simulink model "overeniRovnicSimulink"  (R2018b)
settings: Solver=ode4  StartTime=0.0  StopTime=5  FixedStep=1e-3  RelTol=1e-3
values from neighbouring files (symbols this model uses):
  b_0 = 0    [mainSkript_overeniRovnic.m]    (also in mainSkript_rovniceSystemu.m = (params.bp_0 + params.bn_0) / 2; mainSkript_simulaceLQG.m = (bn_0 + bp_0) / 2; mainSkript_LQGexperiment.m = (bn_0 + bp_0) / 2; mainSkript_LQGexperiment_integral.m = (bn_0 + bp_0) / 2)
  b_1 = params.b_1    [mainSkript_overeniRovnic.m]    (also in mainSkript_rovniceSystemu.m; mainSkript_kyvadlaNajednouOdhad.m; mainSkript_simulaceLQG.m; mainSkript_LQGexperiment.m)
  b_2 = params.b_2    [mainSkript_overeniRovnic.m]    (also in mainSkript_rovniceSystemu.m; mainSkript_kyvadlaNajednouOdhad.m; mainSkript_simulaceLQG.m; mainSkript_LQGexperiment.m)
  dtheta0_0 = 0    [mainSkript_overeniRovnic.m]
  dtheta0_1 = 0    [mainSkript_overeniRovnic.m]    (also in mainSkript_kyvadlaNajednouOdhad.m = filt * dth1(n_start-gl : n_start+gl))
  dtheta0_2 = 0    [mainSkript_overeniRovnic.m]    (also in mainSkript_kyvadlaNajednouOdhad.m = filt * dth2(n_start-gl : n_start+gl))
  g = 9.81    [mainSkript_overeniRovnic.m]    (also in mainSkript_rovniceSystemu.m; mainSkript_estimaceVozik.m; mainSkript_odhadKyvadlaZvlast.m; mainSkript_kyvadlaNajednouOdhad.m)
  I_1 = params.I_1    [mainSkript_overeniRovnic.m]    (also in mainSkript_rovniceSystemu.m; mainSkript_kyvadlaNajednouOdhad.m; mainSkript_simulaceLQG.m; mainSkript_LQGexperiment.m)
  I_2 = params.I_2    [mainSkript_overeniRovnic.m]    (also in mainSkript_rovniceSystemu.m; mainSkript_kyvadlaNajednouOdhad.m; mainSkript_simulaceLQG.m; mainSkript_LQGexperiment.m)
  L_1 = params.L_1    [mainSkript_overeniRovnic.m]    (also in mainSkript_rovniceSystemu.m; odhadovane_parametry.m = 0.228; mainSkript_kyvadlaNajednouOdhad.m; mainSkript_simulaceLQG.m)
  l_1 = params.l_1    [mainSkript_overeniRovnic.m]    (also in mainSkript_rovniceSystemu.m; odhadovane_parametry.m = 0.134; mainSkript_kyvadlaNajednouOdhad.m; mainSkript_simulaceLQG.m)
  l_2 = params.l_2    [mainSkript_overeniRovnic.m]    (also in mainSkript_rovniceSystemu.m; odhadovane_parametry.m = 0.112; mainSkript_kyvadlaNajednouOdhad.m; mainSkript_simulaceLQG.m)
  m = params.m_0    [mainSkript_estimaceVozik.m]    (also in mainSkript_odhadKyvadlaZvlast.m = params.m_2; mainSkript_modifikaceVozik.m = 1.437)
  m_0 = params.m_0    [mainSkript_overeniRovnic.m]    (also in mainSkript_rovniceSystemu.m; mainSkript_simulaceLQG.m; mainSkript_LQGexperiment.m; mainSkript_LQGexperiment_integral.m)
  m_1 = params.m_1    [mainSkript_overeniRovnic.m]    (also in mainSkript_rovniceSystemu.m; mainSkript_kyvadlaNajednouOdhad.m; mainSkript_simulaceLQG.m; mainSkript_LQGexperiment.m)
  m_2 = params.m_2    [mainSkript_overeniRovnic.m]    (also in mainSkript_rovniceSystemu.m; mainSkript_kyvadlaNajednouOdhad.m; mainSkript_simulaceLQG.m; mainSkript_LQGexperiment.m)
  N = N * Cref'    [mainSkript_simulaceLQG.m]    (also in mainSkript_tvorbaTrajektorii.m = 100; mainSkript_pocitaniTVLQR_simplified.m = floor( length(time) / krok ))
  theta0_0 = 0    [mainSkript_overeniRovnic.m]
  theta0_1 = 0.1    [mainSkript_overeniRovnic.m]
  theta0_2 = -0.6    [mainSkript_overeniRovnic.m]
undefined symbols (not defined in the file or in its folder): deg, DiscIntNeverNeededParam, kg, rad, s
libraries: mblibv1 x33, simulink x2
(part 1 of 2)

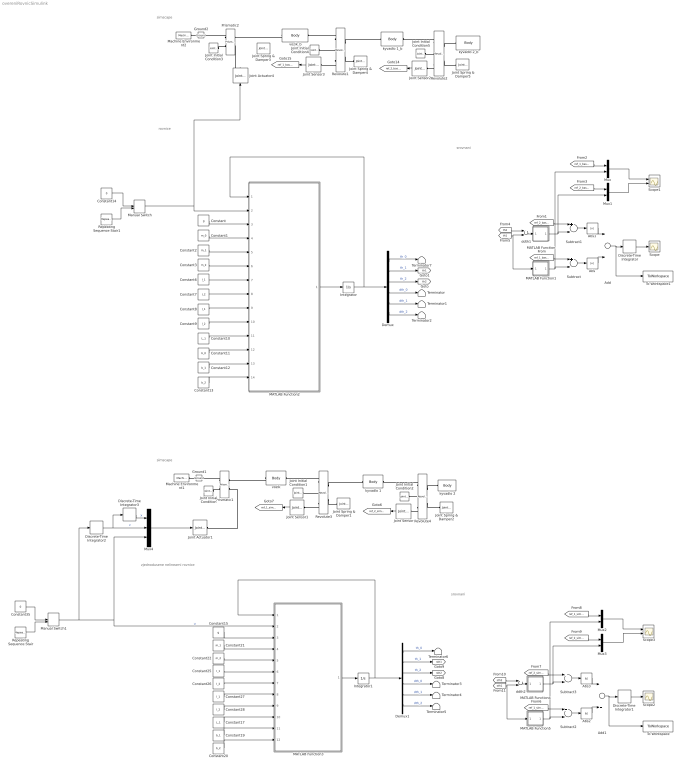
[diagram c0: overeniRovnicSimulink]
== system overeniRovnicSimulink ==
  note: zjednodusene nelinearni rovnice
  note: rovnice
  note: simscape
  note: srovnani
  note: srovnani
  note: simscape
  Abs{,1..3} (4 alike) : Abs
  Add : Sum
  Add1 : Sum
  Constant : Constant  Value=g
  Constant1 : Constant  Value=m_0
  Constant10 : Constant  Value=L_1
  Constant11 : Constant  Value=b_0
  Constant12 : Constant  Value=b_1
  Constant13 : Constant  Value=b_2
  Constant14 : Constant  Value=0
  Constant15 : Constant  Value=g
  Constant17 : Constant  Value=L_1
  Constant19 : Constant  Value=b_1
  Constant2 : Constant  Value=m_1
  Constant20 : Constant  Value=b_2
  Constant21 : Constant  Value=m_1
  Constant22 : Constant  Value=m_2
  Constant25 : Constant  Value=I_1
  Constant26 : Constant  Value=I_2
  Constant27 : Constant  Value=l_1
  Constant28 : Constant  Value=l_2
  Constant3 : Constant  Value=m_2
  Constant35 : Constant  Value=0
  Constant6 : Constant  Value=I_1
  Constant7 : Constant  Value=I_2
  Constant8 : Constant  Value=l_1
  Constant9 : Constant  Value=l_2
  Demux : Demux  Outputs=6
  Demux1 : Demux  Outputs=6
  Discrete-Time Integrator{,1..3} (4 alike) : DiscreteIntegrator  SampleTime=1e-3  ICPrevOutput=DiscIntNeverNeededParam  ICPrevScaledInput=DiscIntNeverNeededParam
  Ground1 : mblibv1/Bodies/Ground  UpdateFromCAD=off  LeftPortType=env  RightPortType=workingframe  PhysicalDomain=Mechanical  DialogClass=GroundBlock  CoordPosition=[0 0 0]  CoordPositionUnits=m  StateVectorMgrId=-1  MachineId=[0 0]  ShowEnvPort=on  ParameterChecksum=[1731498079, 3636340835, 3655824204, 100592062]  TopologyChecksum=[3274135082, 1712955816, 1157478112, 3607701974]
  Ground2 : mblibv1/Bodies/Ground  UpdateFromCAD=off  LeftPortType=env  RightPortType=workingframe  PhysicalDomain=Mechanical  DialogClass=GroundBlock  CoordPosition=[0 0 0]  CoordPositionUnits=m  StateVectorMgrId=-1  MachineId=[0 0]  ShowEnvPort=on  ParameterChecksum=[3763866834, 2337324317, 1522709240, 4291601322]  TopologyChecksum=[3204540527, 4191976194, 257722546, 2930277444]
  Integrator : Integrator  InitialCondition=[theta0_0, theta0_1, theta0_2, dtheta0_0, dtheta0_1, dtheta0_2]
  Integrator1 : Integrator  InitialCondition=[theta0_0, theta0_1, theta0_2, dtheta0_0, dtheta0_1, dtheta0_2]
  Joint Actuator1 : mblibv1/Sensors &  Actuators/Joint Actuator  UpdateFromCAD=off  PhysicalDomain=Mechanical  PortType=blob  ActuationStyle=Motion  AngleUnits=rad  ArcVelocityUnits=rad/s  ArcAccelerationUnits=rad/s^2  CoordPositionUnits=m  VelocityUnits=m/s  AccelerationUnits=m/s^2  ForceUnits=N  TorqueUnits=N*m  ActiveIO=on  Width=3  DialogClass=MechanicalActuatorBlock  Primitive=P1  ReferenceFrame=Absolute (World)
  Joint Actuator4 : mblibv1/Sensors &  Actuators/Joint Actuator  UpdateFromCAD=off  PhysicalDomain=Mechanical  PortType=blob  ActuationStyle=Force  AngleUnits=rad  ArcVelocityUnits=rad/s  ArcAccelerationUnits=rad/s^2  CoordPositionUnits=m  VelocityUnits=m/s  AccelerationUnits=m/s^2  ForceUnits=N  TorqueUnits=N*m  ActiveIO=on  Width=1  DialogClass=MechanicalActuatorBlock  Primitive=P1  ReferenceFrame=Absolute (World)
  Joint Initial Condition : mblibv1/Sensors &  Actuators/Joint Initial Condition  UpdateFromCAD=off  LeftPortType=blob  RightPortType=blob  PhysicalDomain=mechanical  DialogClass=InitialConditionBlock  InitialConditions=P1$true$theta0_0$m$deg$dtheta0_0$m/s$deg/s#P2$false$0$m$deg$0$m/s$deg/s#P3$false$0$m$deg$0$m/s$deg/s#R1$false$0$m$deg$0$m/s$deg/s#R2$false$0$m$deg$0$m/s$deg/s#R3$false$0$m$deg$0$m/s$deg/s#S$false$0$m$deg$0$m/s$deg/s  P1PIC=theta0_0  P1VIC=dtheta0_0  P2PIC=0  P2VIC=0  P3PIC=0  P3VIC=0  R1PIC=0  R1VIC=0  R2PIC=0  R2VIC=0  R3PIC=0  R3VIC=0  SPIC=0  SVIC=0
  Joint Initial Condition1 : mblibv1/Sensors &  Actuators/Joint Initial Condition  UpdateFromCAD=off  LeftPortType=blob  RightPortType=blob  PhysicalDomain=mechanical  DialogClass=InitialConditionBlock  InitialConditions=P1$false$th0i$m$deg$dth0i$m/s$deg/s#P2$false$0$m$deg$0$m/s$deg/s#P3$false$0$m$deg$0$m/s$deg/s#R1$true$theta0_1$m$rad$dtheta0_1$m/s$rad/s#R2$false$0$m$deg$0$m/s$deg/s#R3$false$0$m$deg$0$m/s$deg/s#S$false$0$m$deg$0$m/s$deg/s  P1PIC=0  P1VIC=0  P2PIC=0  P2VIC=0  P3PIC=0  P3VIC=0  R1PIC=theta0_1  R1VIC=dtheta0_1  R2PIC=0  R2VIC=0  R3PIC=0  R3VIC=0  SPIC=0  SVIC=0
  Joint Initial Condition2 : mblibv1/Sensors &  Actuators/Joint Initial Condition  UpdateFromCAD=off  LeftPortType=blob  RightPortType=blob  PhysicalDomain=mechanical  DialogClass=InitialConditionBlock  InitialConditions=P1$false$th0i$m$deg$dth0i$m/s$deg/s#P2$false$0$m$deg$0$m/s$deg/s#P3$false$0$m$deg$0$m/s$deg/s#R1$true$theta0_2 - theta0_1$m$rad$dtheta0_2 - dtheta0_1$m/s$rad/s#R2$false$0$m$deg$0$m/s$deg/s#R3$false$0$m$deg$0$m/s$deg/s#S$false$0$m$deg$0$m/s$deg/s  P1PIC=0  P1VIC=0  P2PIC=0  P2VIC=0  P3PIC=0  P3VIC=0  R1PIC=theta0_2 - theta0_1  R1VIC=dtheta0_2 - dtheta0_1  R2PIC=0  R2VIC=0  R3PIC=0  R3VIC=0  SPIC=0  SVIC=0
  Joint Initial Condition3 : mblibv1/Sensors &  Actuators/Joint Initial Condition  UpdateFromCAD=off  LeftPortType=blob  RightPortType=blob  PhysicalDomain=mechanical  DialogClass=InitialConditionBlock  InitialConditions=P1$true$theta0_0$m$deg$dtheta0_0$m/s$deg/s#P2$false$0$m$deg$0$m/s$deg/s#P3$false$0$m$deg$0$m/s$deg/s#R1$false$0$m$deg$0$m/s$deg/s#R2$false$0$m$deg$0$m/s$deg/s#R3$false$0$m$deg$0$m/s$deg/s#S$false$0$m$deg$0$m/s$deg/s  P1PIC=theta0_0  P1VIC=dtheta0_0  P2PIC=0  P2VIC=0  P3PIC=0  P3VIC=0  R1PIC=0  R1VIC=0  R2PIC=0  R2VIC=0  R3PIC=0  R3VIC=0  SPIC=0  SVIC=0
  Joint Initial Condition4 : mblibv1/Sensors &  Actuators/Joint Initial Condition  UpdateFromCAD=off  LeftPortType=blob  RightPortType=blob  PhysicalDomain=mechanical  DialogClass=InitialConditionBlock  InitialConditions=P1$false$th0i$m$deg$dth0i$m/s$deg/s#P2$false$0$m$deg$0$m/s$deg/s#P3$false$0$m$deg$0$m/s$deg/s#R1$true$theta0_1$m$rad$dtheta0_1$m/s$rad/s#R2$false$0$m$deg$0$m/s$deg/s#R3$false$0$m$deg$0$m/s$deg/s#S$false$0$m$deg$0$m/s$deg/s  P1PIC=0  P1VIC=0  P2PIC=0  P2VIC=0  P3PIC=0  P3VIC=0  R1PIC=theta0_1  R1VIC=dtheta0_1  R2PIC=0  R2VIC=0  R3PIC=0  R3VIC=0  SPIC=0  SVIC=0
  Joint Initial Condition5 : mblibv1/Sensors &  Actuators/Joint Initial Condition  UpdateFromCAD=off  LeftPortType=blob  RightPortType=blob  PhysicalDomain=mechanical  DialogClass=InitialConditionBlock  InitialConditions=P1$false$th0i$m$deg$dth0i$m/s$deg/s#P2$false$0$m$deg$0$m/s$deg/s#P3$false$0$m$deg$0$m/s$deg/s#R1$true$theta0_2 - theta0_1$m$rad$dtheta0_2 - dtheta0_1$m/s$rad/s#R2$false$0$m$deg$0$m/s$deg/s#R3$false$0$m$deg$0$m/s$deg/s#S$false$0$m$deg$0$m/s$deg/s  P1PIC=0  P1VIC=0  P2PIC=0  P2VIC=0  P3PIC=0  P3VIC=0  R1PIC=theta0_2 - theta0_1  R1VIC=dtheta0_2 - dtheta0_1  R2PIC=0  R2VIC=0  R3PIC=0  R3VIC=0  SPIC=0  SVIC=0
  Joint Sensor{,1..3} (4 alike) : mblibv1/Sensors &  Actuators/Joint Sensor  UpdateFromCAD=off  PhysicalDomain=Mechanical  PortType=blob  Muxed=on  Pose=off  Angle=on  AngleUnits=rad  ArcVelocity=off  ArcVelocityUnits=deg/s  ArcAcceleration=off  ArcAccelerationUnits=deg/s^2  CoordPosition=on  CoordPositionUnits=m  Velocity=off  VelocityUnits=m/s  Acceleration=off  AccelerationUnits=m/s^2  Quaternion=on  QuaternionDT=off  QuaternionDDT=off  QuaternionUnits=off  OutputVector=[1]  ActiveIO=on  Width=1  DialogClass=MechanicalSensorBlock  Primitive=R1  Force=off  ForceUnits=N  Torque=off  TorqueUnits=N*m  ReferenceFrame=Absolute (World)  ReactionSensedSide=Base  ReactionReferenceFrame=Absolute (World)  ReactionForce=off  ReactionForceUnits=N  ReactionMoment=off  ReactionMomentUnits=N*m
  Joint Spring & Damper1 : mblibv1/Force  Elements/Joint Spring & Damper  UpdateFromCAD=off  DialogClass=JointSpringDamper  JFEParameters=P1$false$0$b0$0$m$m/s$N$deg$deg/s$N*m#P2$false$0$0$0$m$m/s$N$deg$deg/s$N*m#P3$false$0$0$0$m$m/s$N$deg$deg/s$N*m#R1$true$0$b_1$0$m$m/s$N$rad$rad/s$N*m#R2$false$0$0$0$m$m/s$N$deg$deg/s$N*m#R3$false$0$0$0$m$m/s$N$deg$deg/s$N*m#S$false$0$0$0$m$m/s$N$deg$deg/s$N*m
  Joint Spring & Damper2 : mblibv1/Force  Elements/Joint Spring & Damper  UpdateFromCAD=off  DialogClass=JointSpringDamper  JFEParameters=P1$false$0$b0$0$m$m/s$N$deg$deg/s$N*m#P2$false$0$0$0$m$m/s$N$deg$deg/s$N*m#P3$false$0$0$0$m$m/s$N$deg$deg/s$N*m#R1$true$0$b_2$0$m$m/s$N$rad$rad/s$N*m#R2$false$0$0$0$m$m/s$N$deg$deg/s$N*m#R3$false$0$0$0$m$m/s$N$deg$deg/s$N*m#S$false$0$0$0$m$m/s$N$deg$deg/s$N*m
  Joint Spring & Damper3 : mblibv1/Force  Elements/Joint Spring & Damper  UpdateFromCAD=off  DialogClass=JointSpringDamper  JFEParameters=P1$true$0$b_0$0$m$m/s$N$deg$deg/s$N*m#P2$false$0$0$0$m$m/s$N$deg$deg/s$N*m#P3$false$0$0$0$m$m/s$N$deg$deg/s$N*m#R1$false$0$0$0$m$m/s$N$deg$deg/s$N*m#R2$false$0$0$0$m$m/s$N$deg$deg/s$N*m#R3$false$0$0$0$m$m/s$N$deg$deg/s$N*m#S$false$0$0$0$m$m/s$N$deg$deg/s$N*m
  Joint Spring & Damper4 : mblibv1/Force  Elements/Joint Spring & Damper  UpdateFromCAD=off  DialogClass=JointSpringDamper  JFEParameters=P1$false$0$b0$0$m$m/s$N$deg$deg/s$N*m#P2$false$0$0$0$m$m/s$N$deg$deg/s$N*m#P3$false$0$0$0$m$m/s$N$deg$deg/s$N*m#R1$true$0$b_1$0$m$m/s$N$rad$rad/s$N*m#R2$false$0$0$0$m$m/s$N$deg$deg/s$N*m#R3$false$0$0$0$m$m/s$N$deg$deg/s$N*m#S$false$0$0$0$m$m/s$N$deg$deg/s$N*m
  Joint Spring & Damper5 : mblibv1/Force  Elements/Joint Spring & Damper  UpdateFromCAD=off  DialogClass=JointSpringDamper  JFEParameters=P1$false$0$b0$0$m$m/s$N$deg$deg/s$N*m#P2$false$0$0$0$m$m/s$N$deg$deg/s$N*m#P3$false$0$0$0$m$m/s$N$deg$deg/s$N*m#R1$true$0$b_2$0$m$m/s$N$rad$rad/s$N*m#R2$false$0$0$0$m$m/s$N$deg$deg/s$N*m#R3$false$0$0$0$m$m/s$N$deg$deg/s$N*m#S$false$0$0$0$m$m/s$N$deg$deg/s$N*m
  MATLAB Function : MATLAB Function  TreatAsAtomicUnit=on
  MATLAB Function1 : MATLAB Function  TreatAsAtomicUnit=on
  MATLAB Function2 : MATLAB Function  TreatAsAtomicUnit=on
  MATLAB Function3 : MATLAB Function  TreatAsAtomicUnit=on
  MATLAB Function4 : MATLAB Function  TreatAsAtomicUnit=on
  MATLAB Function5 : MATLAB Function  TreatAsAtomicUnit=on
  Machine Environment1 : mblibv1/Bodies/Machine Environment  PortType=env  PhysicalDomain=Mechanical  DialogTemplateClass=MECH.MachineEnvironment  SyncWhenCopied=off  Gravity=[0 -g 0]  GravityUnits=m/s^2  GravityAsSignal=off  Dimensionality=Auto-detect  AnalysisType=Forward dynamics  LinearAssemblyTolerance=1e-3  LinearAssemblyToleranceUnits=m  AngularAssemblyTolerance=1e-3  AngularAssemblyToleranceUnits=rad  ConstraintSolverType=Stabilizing  ConstraintRelTolerance=1e-4  ConstraintAbsTolerance=1e-4  UseRobustSingularityHandling=off  RedundancyAnalysisToleranceType=Automatically select tolerance  RedundancyAnalysisTolerance=1e-14  StatePerturbationType=Fixed  PerturbationSize=1e-5  VisualizeMachine=on  BodyVisualizationType=Use model default body geometries  BodyColorSelMode=Use model default  DefaultBodyColor=[1 0 0]
  Machine Environment2 : mblibv1/Bodies/Machine Environment  PortType=env  PhysicalDomain=Mechanical  DialogTemplateClass=MECH.MachineEnvironment  SyncWhenCopied=off  Gravity=[0 -g 0]  GravityUnits=m/s^2  GravityAsSignal=off  Dimensionality=Auto-detect  AnalysisType=Forward dynamics  LinearAssemblyTolerance=1e-3  LinearAssemblyToleranceUnits=m  AngularAssemblyTolerance=1e-3  AngularAssemblyToleranceUnits=rad  ConstraintSolverType=Stabilizing  ConstraintRelTolerance=1e-4  ConstraintAbsTolerance=1e-4  UseRobustSingularityHandling=off  RedundancyAnalysisToleranceType=Automatically select tolerance  RedundancyAnalysisTolerance=1e-14  StatePerturbationType=Fixed  PerturbationSize=1e-5  VisualizeMachine=on  BodyVisualizationType=Use model default body geometries  BodyColorSelMode=Use model default  DefaultBodyColor=[1 0 0]
  Manual Switch : ManualSwitch  CurrentSetting=0
  Manual Switch1 : ManualSwitch  CurrentSetting=0
  Mux{,1..3} (4 alike) : Mux  Inputs=2
  Mux4 : Mux  Inputs=3
  Prismatic1 : mblibv1/Joints/Prismatic  LConnTagsString=__newl0|SA1  RConnTagsString=__newr0|SA1  UpdateFromCAD=off  NumSAPorts=2  CutJoint=off  MarkAsCut=off  Primitives=prismatic  PrimitiveProps=P1$World$[-1 0 0]$prismatic  DialogClass=JointBlock  P1Axis=[-1 0 0]
  Prismatic2 : mblibv1/Joints/Prismatic  LConnTagsString=__newl0|SA1  RConnTagsString=__newr0|SA1  UpdateFromCAD=off  NumSAPorts=2  CutJoint=off  MarkAsCut=off  Primitives=prismatic  PrimitiveProps=P1$World$[-1 0 0]$prismatic  DialogClass=JointBlock  P1Axis=[-1 0 0]
  Repeating Sequence Stair : simulink/Sources/Repeating Sequence Stair  OutValues=[3 -3 2 -2 0].'  tsamp=-1  OutMin=[]  OutMax=[]  OutDataTypeStr=double  OutputDataTypeScalingMode=double  OutDataType=fixdt(0,8)  ConRadixGroup=Best Precision: Vector-wise  OutScaling=2^-12
  Repeating Sequence Stair1 : simulink/Sources/Repeating Sequence Stair  OutValues=[3 -3 2 -2 0].'  tsamp=-1  OutMin=[]  OutMax=[]  OutDataTypeStr=double  OutputDataTypeScalingMode=double  OutDataType=fixdt(0,8)  ConRadixGroup=Best Precision: Vector-wise  OutScaling=2^-12
  Revolute1 : mblibv1/Joints/Revolute  LConnTagsString=__newl0|SA1|SA2  RConnTagsString=__newr0|SA1  UpdateFromCAD=off  NumSAPorts=3  CutJoint=off  MarkAsCut=off  Primitives=prismatic  PrimitiveProps=R1$World$[0 0 1]$revolute  DialogClass=JointBlock  R1Axis=[0 0 1]
  Revolute2 : mblibv1/Joints/Revolute  LConnTagsString=__newl0|SA1|SA2  RConnTagsString=__newr0|SA1  UpdateFromCAD=off  NumSAPorts=3  CutJoint=off  MarkAsCut=off  Primitives=prismatic  PrimitiveProps=R1$Base$[0 0 1]$revolute  DialogClass=JointBlock  R1Axis=[0 0 1]
  Revolute3 : mblibv1/Joints/Revolute  LConnTagsString=__newl0|SA1|SA2  RConnTagsString=__newr0|SA1  UpdateFromCAD=off  NumSAPorts=3  CutJoint=off  MarkAsCut=off  Primitives=prismatic  PrimitiveProps=R1$World$[0 0 1]$revolute  DialogClass=JointBlock  R1Axis=[0 0 1]
  Revolute4 : mblibv1/Joints/Revolute  LConnTagsString=__newl0|SA1|SA2  RConnTagsString=__newr0|SA1  UpdateFromCAD=off  NumSAPorts=3  CutJoint=off  MarkAsCut=off  Primitives=prismatic  PrimitiveProps=R1$Base$[0 0 1]$revolute  DialogClass=JointBlock  R1Axis=[0 0 1]
  Scope : Scope
  Scope1 : Scope  NumInputPorts=2
  Scope2 : Scope
  Scope3 : Scope  NumInputPorts=2
  Subtract{,1..3} (4 alike) : Sum  Inputs=+-
  Terminator{,1..7} (8 alike) : Terminator
  To Workspace : ToWorkspace  VariableName=odchylka_simplified  SaveFormat=Structure With Time  SampleTime=-1
  To Workspace1 : ToWorkspace  VariableName=odchylka_basic  SaveFormat=Structure With Time  SampleTime=-1
  ddth1 : Sum  Inputs=+-
  ddth2 : Sum  Inputs=+-
  kyvadlo 1 : mblibv1/Bodies/Body  LConnTagsString=CS1  RConnTagsString=CS2  UpdateFromCAD=off  DialogClass=MechanicalBodyBlock  Mass=m_1  MassUnits=kg  InertiaUnits=kg*m^2  Inertia=eye(3)*I_1  Shape=Cylinder  ShapeDims=[1 1]  ShapeUnits=m  ShapeUse=false  Density=1  DensityUnits=kg/m^3  DensityUse=false  GraphicsMode=MACHINE_DEFAULT  BodyColorSelMode=COLORPALETTE  BodyColor=[0 0 0]  AttachedToCS=CG  CG=Left$CG$[0 l_1 0]$CS1$CS1$m$[0 0 0]$Euler X-Y-Z$deg$WORLD$false$none  WorkingFrames=Left$CS1$[0 0 0]$Adjoining$Adjoining$m$[0 0 0]$Euler X-Y-Z$deg$WORLD$true$none#Right$CS2$[0 L_1 0]$CS1$CS1$m$[0 0 0]$Euler X-Y-Z$deg$WORLD$true$none  CGPos=[0 l_1 0]  CGRot=[0 0 0]  CS0Pos=[]  CS0Rot=[]  CS1Pos=[0 0 0]  CS1Rot=[0 0 0]  CS2Pos=[0 L_1 0]  CS2Rot=[0 0 0]  CS3Pos=[]  CS3Rot=[]  CS4Pos=[]  CS4Rot=[]  CS5Pos=[]  CS5Rot=[]  CS6Pos=[]  CS6Rot=[]  CS7Pos=[]  CS7Rot=[]  CS8Pos=[]  CS8Rot=[]  CS9Pos=[]  CS9Rot=[]  CS10Pos=[]  CS10Rot=[]  CS11Pos=[]  CS11Rot=[]  CS12Pos=[]  CS12Rot=[]  CS13Pos=[]  CS13Rot=[]  CS14Pos=[]  CS14Rot=[]  CS15Pos=[]  CS15Rot=[]  CS16Pos=[]  CS16Rot=[]  CS17Pos=[]  CS17Rot=[]  CS18Pos=[]  CS18Rot=[]  CS19Pos=[]  CS19Rot=[]  CS20Pos=[]  CS20Rot=[]
  kyvadlo 1_b : mblibv1/Bodies/Body  LConnTagsString=CS1  RConnTagsString=CS2  UpdateFromCAD=off  DialogClass=MechanicalBodyBlock  Mass=m_1  MassUnits=kg  InertiaUnits=kg*m^2  Inertia=eye(3)*I_1  Shape=Cylinder  ShapeDims=[1 1]  ShapeUnits=m  ShapeUse=false  Density=1  DensityUnits=kg/m^3  DensityUse=false  GraphicsMode=MACHINE_DEFAULT  BodyColorSelMode=COLORPALETTE  BodyColor=[0 0 0]  AttachedToCS=CG  CG=Left$CG$[0 l_1 0]$CS1$CS1$m$[0 0 0]$Euler X-Y-Z$deg$WORLD$false$none  WorkingFrames=Left$CS1$[0 0 0]$Adjoining$Adjoining$m$[0 0 0]$Euler X-Y-Z$deg$WORLD$true$none#Right$CS2$[0 L_1 0]$CS1$CS1$m$[0 0 0]$Euler X-Y-Z$deg$WORLD$true$none  CGPos=[0 l_1 0]  CGRot=[0 0 0]  CS0Pos=[]  CS0Rot=[]  CS1Pos=[0 0 0]  CS1Rot=[0 0 0]  CS2Pos=[0 L_1 0]  CS2Rot=[0 0 0]  CS3Pos=[]  CS3Rot=[]  CS4Pos=[]  CS4Rot=[]  CS5Pos=[]  CS5Rot=[]  CS6Pos=[]  CS6Rot=[]  CS7Pos=[]  CS7Rot=[]  CS8Pos=[]  CS8Rot=[]  CS9Pos=[]  CS9Rot=[]  CS10Pos=[]  CS10Rot=[]  CS11Pos=[]  CS11Rot=[]  CS12Pos=[]  CS12Rot=[]  CS13Pos=[]  CS13Rot=[]  CS14Pos=[]  CS14Rot=[]  CS15Pos=[]  CS15Rot=[]  CS16Pos=[]  CS16Rot=[]  CS17Pos=[]  CS17Rot=[]  CS18Pos=[]  CS18Rot=[]  CS19Pos=[]  CS19Rot=[]  CS20Pos=[]  CS20Rot=[]
  kyvadlo 2 : mblibv1/Bodies/Body  LConnTagsString=CS1  RConnTagsString=CS2  UpdateFromCAD=off  DialogClass=MechanicalBodyBlock  Mass=m_2  MassUnits=kg  InertiaUnits=kg*m^2  Inertia=eye(3)*I_2  Shape=Cylinder  ShapeDims=[1 1]  ShapeUnits=m  ShapeUse=false  Density=1  DensityUnits=kg/m^3  DensityUse=false  GraphicsMode=MACHINE_DEFAULT  BodyColorSelMode=COLORPALETTE  BodyColor=[0 0 0]  AttachedToCS=CG  CG=Left$CG$[0 l_2 0]$CS1$CS1$m$[0 0 0]$Euler X-Y-Z$deg$WORLD$false$none  WorkingFrames=Left$CS1$[0 0 0]$Adjoining$Adjoining$m$[0 0 0]$Euler X-Y-Z$deg$WORLD$true$none#Right$CS2$[0 2*l_2 0]$CS1$CS1$m$[0 0 0]$Euler X-Y-Z$deg$WORLD$true$none  CGPos=[0 l_2 0]  CGRot=[0 0 0]  CS0Pos=[]  CS0Rot=[]  CS1Pos=[0 0 0]  CS1Rot=[0 0 0]  CS2Pos=[0 2*l_2 0]  CS2Rot=[0 0 0]  CS3Pos=[]  CS3Rot=[]  CS4Pos=[]  CS4Rot=[]  CS5Pos=[]  CS5Rot=[]  CS6Pos=[]  CS6Rot=[]  CS7Pos=[]  CS7Rot=[]  CS8Pos=[]  CS8Rot=[]  CS9Pos=[]  CS9Rot=[]  CS10Pos=[]  CS10Rot=[]  CS11Pos=[]  CS11Rot=[]  CS12Pos=[]  CS12Rot=[]  CS13Pos=[]  CS13Rot=[]  CS14Pos=[]  CS14Rot=[]  CS15Pos=[]  CS15Rot=[]  CS16Pos=[]  CS16Rot=[]  CS17Pos=[]  CS17Rot=[]  CS18Pos=[]  CS18Rot=[]  CS19Pos=[]  CS19Rot=[]  CS20Pos=[]  CS20Rot=[]
  kyvadlo 2_b : mblibv1/Bodies/Body  LConnTagsString=CS1  RConnTagsString=CS2  UpdateFromCAD=off  DialogClass=MechanicalBodyBlock  Mass=m_2  MassUnits=kg  InertiaUnits=kg*m^2  Inertia=eye(3)*I_2  Shape=Cylinder  ShapeDims=[1 1]  ShapeUnits=m  ShapeUse=false  Density=1  DensityUnits=kg/m^3  DensityUse=false  GraphicsMode=MACHINE_DEFAULT  BodyColorSelMode=COLORPALETTE  BodyColor=[0 0 0]  AttachedToCS=CG  CG=Left$CG$[0 l_2 0]$CS1$CS1$m$[0 0 0]$Euler X-Y-Z$deg$WORLD$false$none  WorkingFrames=Left$CS1$[0 0 0]$Adjoining$Adjoining$m$[0 0 0]$Euler X-Y-Z$deg$WORLD$true$none#Right$CS2$[0 2*l_2 0]$CS1$CS1$m$[0 0 0]$Euler X-Y-Z$deg$WORLD$true$none  CGPos=[0 l_2 0]  CGRot=[0 0 0]  CS0Pos=[]  CS0Rot=[]  CS1Pos=[0 0 0]  CS1Rot=[0 0 0]  CS2Pos=[0 2*l_2 0]  CS2Rot=[0 0 0]  CS3Pos=[]  CS3Rot=[]  CS4Pos=[]  CS4Rot=[]  CS5Pos=[]  CS5Rot=[]  CS6Pos=[]  CS6Rot=[]  CS7Pos=[]  CS7Rot=[]  CS8Pos=[]  CS8Rot=[]  CS9Pos=[]  CS9Rot=[]  CS10Pos=[]  CS10Rot=[]  CS11Pos=[]  CS11Rot=[]  CS12Pos=[]  CS12Rot=[]  CS13Pos=[]  CS13Rot=[]  CS14Pos=[]  CS14Rot=[]  CS15Pos=[]  CS15Rot=[]  CS16Pos=[]  CS16Rot=[]  CS17Pos=[]  CS17Rot=[]  CS18Pos=[]  CS18Rot=[]  CS19Pos=[]  CS19Rot=[]  CS20Pos=[]  CS20Rot=[]
  vozik_b : mblibv1/Bodies/Body  LConnTagsString=CS1  RConnTagsString=CS2  UpdateFromCAD=off  DialogClass=MechanicalBodyBlock  Mass=m_0  MassUnits=kg  InertiaUnits=kg*m^2  Inertia=zeros(3)  Shape=Cylinder  ShapeDims=[1 1]  ShapeUnits=m  ShapeUse=false  Density=1  DensityUnits=kg/m^3  DensityUse=false  GraphicsMode=MACHINE_DEFAULT  BodyColorSelMode=COLORPALETTE  BodyColor=[0 0 0]  AttachedToCS=CG  CG=Left$CG$[0 0 0]$WORLD$WORLD$m$[0 0 0]$Euler X-Y-Z$deg$WORLD$false$none  WorkingFrames=Left$CS1$[0 0 0]$CG$CG$m$[0 0 0]$Euler X-Y-Z$deg$WORLD$true$none#Right$CS2$[0 0 0]$CG$CG$m$[0 0 0]$Euler X-Y-Z$deg$WORLD$true$none  CGPos=[0 0 0]  CGRot=[0 0 0]  CS0Pos=[]  CS0Rot=[]  CS1Pos=[0 0 0]  CS1Rot=[0 0 0]  CS2Pos=[0 0 0]  CS2Rot=[0 0 0]  CS3Pos=[]  CS3Rot=[]  CS4Pos=[]  CS4Rot=[]  CS5Pos=[]  CS5Rot=[]  CS6Pos=[]  CS6Rot=[]  CS7Pos=[]  CS7Rot=[]  CS8Pos=[]  CS8Rot=[]  CS9Pos=[]  CS9Rot=[]  CS10Pos=[]  CS10Rot=[]  CS11Pos=[]  CS11Rot=[]  CS12Pos=[]  CS12Rot=[]  CS13Pos=[]  CS13Rot=[]  CS14Pos=[]  CS14Rot=[]  CS15Pos=[]  CS15Rot=[]  CS16Pos=[]  CS16Rot=[]  CS17Pos=[]  CS17Rot=[]  CS18Pos=[]  CS18Rot=[]  CS19Pos=[]  CS19Rot=[]  CS20Pos=[]  CS20Rot=[]
  vozík : mblibv1/Bodies/Body  LConnTagsString=CS1  RConnTagsString=CS2  UpdateFromCAD=off  DialogClass=MechanicalBodyBlock  Mass=m_0  MassUnits=kg  InertiaUnits=kg*m^2  Inertia=zeros(3)  Shape=Cylinder  ShapeDims=[1 1]  ShapeUnits=m  ShapeUse=false  Density=1  DensityUnits=kg/m^3  DensityUse=false  GraphicsMode=MACHINE_DEFAULT  BodyColorSelMode=COLORPALETTE  BodyColor=[0 0 0]  AttachedToCS=CG  CG=Left$CG$[0 0 0]$WORLD$WORLD$m$[0 0 0]$Euler X-Y-Z$deg$WORLD$false$none  WorkingFrames=Left$CS1$[0 0 0]$CG$CG$m$[0 0 0]$Euler X-Y-Z$deg$WORLD$true$none#Right$CS2$[0 0 0]$CG$CG$m$[0 0 0]$Euler X-Y-Z$deg$WORLD$true$none  CGPos=[0 0 0]  CGRot=[0 0 0]  CS0Pos=[]  CS0Rot=[]  CS1Pos=[0 0 0]  CS1Rot=[0 0 0]  CS2Pos=[0 0 0]  CS2Rot=[0 0 0]  CS3Pos=[]  CS3Rot=[]  CS4Pos=[]  CS4Rot=[]  CS5Pos=[]  CS5Rot=[]  CS6Pos=[]  CS6Rot=[]  CS7Pos=[]  CS7Rot=[]  CS8Pos=[]  CS8Rot=[]  CS9Pos=[]  CS9Rot=[]  CS10Pos=[]  CS10Rot=[]  CS11Pos=[]  CS11Rot=[]  CS12Pos=[]  CS12Rot=[]  CS13Pos=[]  CS13Rot=[]  CS14Pos=[]  CS14Rot=[]  CS15Pos=[]  CS15Rot=[]  CS16Pos=[]  CS16Rot=[]  CS17Pos=[]  CS17Rot=[]  CS18Pos=[]  CS18Rot=[]  CS19Pos=[]  CS19Rot=[]  CS20Pos=[]  CS20Rot=[]
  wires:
  Add/1 -> To Workspace1/1, Discrete-Time Integrator/1
  Subtract/1 -> Abs/1
  Abs/1 -> Add/2
  [th2] -> ddth1/1
  Abs1/1 -> Add/1
  Subtract1/1 -> Abs1/1
  [th1] -> MATLAB Function1/1(u), ddth1/2
  ddth1/1 -> MATLAB Function/1(u)
  Discrete-Time Integrator/1 -> Scope/1
  Constant2/1 -> MATLAB Function2/5(m_1)
  Constant3/1 -> MATLAB Function2/6(m_2)
  MATLAB Function2/1(dx) -> Integrator/1
  Constant6/1 -> MATLAB Function2/7(I_1)
  Demux/3 -> [th2]  "th_2"
  Constant8/1 -> MATLAB Function2/9(l_1)
  Constant9/1 -> MATLAB Function2/10(l_2)
  Constant12/1 -> MATLAB Function2/13(b_1)
  Demux/2 -> [th1]  "th_1"
  Constant7/1 -> MATLAB Function2/8(I_2)
  Constant11/1 -> MATLAB Function2/12(b_0)
  Constant/1 -> MATLAB Function2/3(g)
  Constant10/1 -> MATLAB Function2/11(L_1)
  Integrator/1 -> MATLAB Function2/1(y), Demux/1
  Constant13/1 -> MATLAB Function2/14(b_2)
  Constant1/1 -> MATLAB Function2/4(m_0)
  Mux/1 -> Scope1/1
  Mux1/1 -> Scope1/2
  Demux/1 -> Terminator7/1  "th_0"
  Demux/4 -> Terminator/1  "dth_0"
  Demux/6 -> Terminator2/1  "dth_2"
  Demux/5 -> Terminator1/1  "dth_1"
  Joint Sensor/1 -> [ref_2_simpl]
  Joint Sensor1/1 -> [ref_1_simpl]
  [ref_1_basic] -> Subtract/1
  [ref_2_basic] -> Subtract1/1
  [ref_1_basic] -> Mux/1
  [ref_2_basic] -> Mux1/1
  MATLAB Function/1(y) -> Mux1/2, Subtract1/2
  MATLAB Function1/1(y) -> Mux/2, Subtract/2
  Constant14/1 -> Manual Switch/1
  Manual Switch/1 -> Joint Actuator4/1, MATLAB Function2/2(u)
  Constant19/1 -> MATLAB Function3/11(b_1)
  Constant20/1 -> MATLAB Function3/12(b_2)
  Constant28/1 -> MATLAB Function3/9(l_2)
  Constant27/1 -> MATLAB Function3/8(l_1)
  Constant17/1 -> MATLAB Function3/10(L_1)
  Constant25/1 -> MATLAB Function3/6(I_1)
  Constant22/1 -> MATLAB Function3/5(m_2)
  Constant26/1 -> MATLAB Function3/7(I_2)
  Constant21/1 -> MATLAB Function3/4(m_1)
  Constant15/1 -> MATLAB Function3/3(g)
  Manual Switch1/1 -> MATLAB Function3/2(u), Mux4/3, Discrete-Time Integrator2/1  "u"
  MATLAB Function3/1(dx) -> Integrator1/1
  Demux1/4 -> Terminator3/1  "dth_0"
  Demux1/6 -> Terminator5/1  "dth_2"
  Demux1/5 -> Terminator4/1  "dth_1"
  Demux1/3 -> [sth2]  "th_2"
  Demux1/2 -> [sth1]  "th_1"
  Demux1/1 -> Terminator6/1  "th_0"
  Integrator1/1 -> Demux1/1, MATLAB Function3/1(y)
  ddth2/1 -> MATLAB Function4/1(u)
  MATLAB Function5/1(y) -> Mux2/2, Subtract2/2
  Abs3/1 -> Add1/1
  [ref_2_simpl] -> Subtract3/1
  Mux3/1 -> Scope3/2
  Abs2/1 -> Add1/2
  [ref_1_simpl] -> Subtract2/1
  MATLAB Function4/1(y) -> Mux3/2, Subtract3/2
  [ref_1_simpl] -> Mux2/1
  Subtract2/1 -> Abs2/1
  [ref_2_simpl] -> Mux3/1
  Mux2/1 -> Scope3/1
  Add1/1 -> To Workspace/1, Discrete-Time Integrator1/1
  [sth2] -> ddth2/1
  Subtract3/1 -> Abs3/1
  [sth1] -> MATLAB Function5/1(u), ddth2/2
  Discrete-Time Integrator1/1 -> Scope2/1
  Discrete-Time Integrator2/1 -> Mux4/2, Discrete-Time Integrator3/1  "v"
  Discrete-Time Integrator3/1 -> Mux4/1  "x"
  Mux4/1 -> Joint Actuator1/1
  Joint Sensor3/1 -> [ref_1_basic]
  Joint Sensor2/1 -> [ref_2_basic]
  Constant35/1 -> Manual Switch1/1
  Repeating Sequence Stair/1 -> Manual Switch1/2
  Repeating Sequence Stair1/1 -> Manual Switch/2
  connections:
  Joint Initial Condition2/RConn1 -- Revolute4/LConn2
  Revolute4/LConn3 -- Joint Sensor/LConn1
  Revolute3/LConn3 -- Joint Sensor1/LConn1
  vozík/LConn1 -- Prismatic1/RConn1
  Joint Initial Condition1/RConn1 -- Revolute3/LConn2
  Prismatic1/LConn1 -- Ground1/RConn1
  Revolute3/RConn1 -- kyvadlo 1/LConn1
  Revolute4/RConn1 -- kyvadlo 2/LConn1
  Revolute3/LConn1 -- vozík/RConn1
  Revolute4/LConn1 -- kyvadlo 1/RConn1
  Revolute3/RConn2 -- Joint Spring & Damper1/LConn1
  Machine Environment1/RConn1 -- Ground1/LConn1
  Revolute4/RConn2 -- Joint Spring & Damper2/LConn1
  Joint Initial Condition/RConn1 -- Prismatic1/LConn2
  Joint Actuator1/RConn1 -- Prismatic1/RConn2
  Machine Environment2/RConn1 -- Ground2/LConn1
  Joint Initial Condition5/RConn1 -- Revolute2/LConn2
  Revolute1/LConn3 -- Joint Sensor3/LConn1
  Revolute1/LConn1 -- vozik_b/RConn1
  Revolute2/RConn1 -- kyvadlo 2_b/LConn1
  Revolute2/RConn2 -- Joint Spring & Damper5/LConn1
  Prismatic2/RConn2 -- Joint Actuator4/RConn1
  Revolute2/LConn1 -- kyvadlo 1_b/RConn1
  Joint Initial Condition3/RConn1 -- Prismatic2/LConn2
  Revolute1/RConn2 -- Joint Spring & Damper4/LConn1
  Joint Initial Condition4/RConn1 -- Revolute1/LConn2
  Revolute1/RConn1 -- kyvadlo 1_b/LConn1
  Prismatic2/LConn1 -- Ground2/RConn1
  Revolute2/LConn3 -- Joint Sensor2/LConn1
  vozik_b/LConn1 -- Prismatic2/RConn1

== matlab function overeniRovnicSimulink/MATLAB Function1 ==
function y = fcn(u)
%#codegen

y = mod(u+pi,2*pi)-pi;

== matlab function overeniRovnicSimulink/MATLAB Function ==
function y = fcn(u)
%#codegen

y = mod(u+pi,2*pi)-pi;
